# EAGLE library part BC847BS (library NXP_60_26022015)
NPN/NPN general-purpose transistor pair in a very small SOT363 (SC-88) Surface-Mounted Device (SMD) plastic package. AAL Eindhoven MK
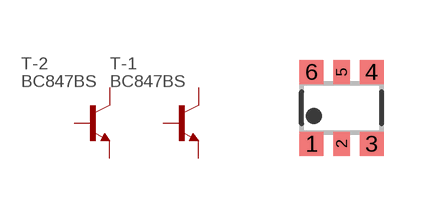
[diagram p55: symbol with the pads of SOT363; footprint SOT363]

Designator prefix T; gates -1=NPN -2=NPN

## BC847BS  [SOT363]
1  -1:E  pas
2  -1:B  pas
3  -2:C  pas
4  -2:E  pas
5  -2:B  pas
6  -1:C  pas

## Footprint SOT363 (pad centres in mm)
SOT363 Plastic surface-mounted package; 6 leads JEDEC: -- IEC: -- JEITA: SC-88
smd 0.6 x 0.6: 1 -0.75,-0.9; 3 0.75,-0.9; 4 0.75,0.9; 6 -0.75,0.9
smd 0.4 x 0.6: 2 0,-0.9; 5 0,0.9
